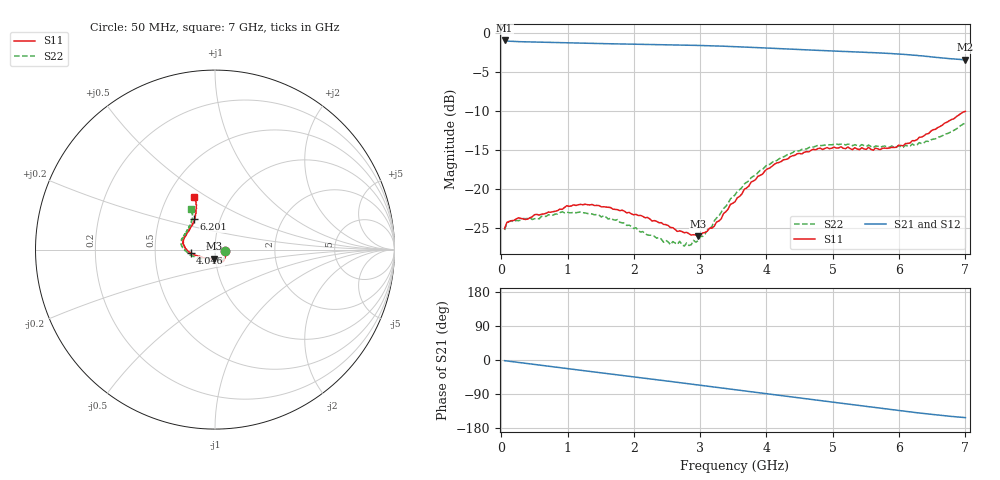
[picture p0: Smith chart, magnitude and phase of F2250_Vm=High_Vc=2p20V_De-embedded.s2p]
! Integrated Device Technology
! Corporate Headquarters
! 6024 Silver Creek Valley Road
! San Jose, CA 95138  USA
! Phone:  1-408-284-8200
! Toll Free:  1-800-223-1366
! Webpage:  http://www.idt.com/
! Timing and RF Division
! 515 Groton Road, Suite 102
! Westford, MA 01886-6024
! Device:  F2250
! Description: Voltage Variable RF Attenuator
! Frequency:  50.0 -  6000.00 MHz
! Package:  3x3 mm Thin QFN Plastic Package: 16 pin
! Ports:  2 RF, 3 DC
!  Pin  1  = GND
!  Pin  2  = NC
!  Pin  3  = RF1  = Port 1
!  Pin  4  = NC
!  Pin  5  = GND
!  Pin  6  = GND
!  Pin  7  = GND
!  Pin  8  = GND
!  Pin  9  = NC
!  Pin 10  = RF2  = Port 2
!  Pin 11  = NC
!  Pin 12  = GND
!  Pin 13  = GND
!  Pin 14  = VCNTRL
!  Pin 15  = VDD
!  Pin 16  = VMODE
! Vcntrl:  2.200 Volts
! Vmode:  +3.300 Volts
! Vdd:  +3.30  Volts
! Current:  1.317 mA
! Data:  The device was measured on a the F2250 evaluation board which has
!  individual transmission lines to the RF pins.  Data was collected
!  using a calibrated network analyzer.  The evaluation board was
!  de-embedded using a TRL calibration technique.
!  The reference plane is the edge of the package pin.
! Misc:  SN 10
!  Action Tracker AT0258
! Date Measured:  2014-11-26
! Date:  2015-10-15  MJV
! Note:
!  Integrated Device Technology supplies this data as a sample of measured
!  data at the package pin for this product.  Your particular data for this
!  product may vary.
!  Data was taken at 25 degrees C.
!  Integrated Device Technology reserves the right to change this data at anytime.
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# GHz S dB R 50
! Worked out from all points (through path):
!   201 points, 50 MHz to 7 GHz, reference 50 ohm
!   highest |S21| = -0.93 dB at 50 MHz (marker M1); lowest = -3.4 dB at 7 GHz (marker M2)
!   group delay of S21, straight-line fit = 61.1 ps
!   lowest |S11| = -26.0 dB at 2.969 GHz (marker M3), VSWR 1.11, Z = 49.4 - j4.96 ohm
!   |S11| at or under -10 dB: start of sweep to end of sweep
!   |S22| runs from -27.3 to -11.5 dB; largest |S21 - S12| = 0.0019
!   S11 on the Smith chart (normalised r, x): 50 MHz: 1.12, -0.02; 4.046 GHz: 0.76, -0.03; 6.201 GHz: 0.75, +0.27; 7 GHz: 0.68, +0.44
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0.05  -25.02 -9.9  -0.93 -1.8  -0.93 -1.8  -25.20 -10.3
0.08475  -24.23 -9.1  -1.00 -2.5  -1.00 -2.5  -24.28 -9.2
0.1195  -24.12 -9.6  -1.03 -3.2  -1.03 -3.2  -24.09 -8.5
0.91875  -22.56 -48.1  -1.21 -21.0  -1.21 -21.1  -22.87 -49.8
1.2315  -21.97 -55.9  -1.28 -27.9  -1.28 -27.9  -22.99 -60.3
1.75275  -22.59 -62.8  -1.37 -39.1  -1.37 -39.1  -23.87 -67.1
2.37825  -24.27 -62.8  -1.46 -52.8  -1.46 -52.8  -26.16 -67.8
2.552  -24.89 -67.4  -1.49 -56.6  -1.49 -56.7  -27.08 -74.4
2.691  -25.31 -75.0  -1.51 -59.7  -1.51 -59.8  -26.65 -81.7
2.7605  -25.55 -77.0  -1.53 -61.3  -1.53 -61.3  -27.27 -86.1
2.969  -25.99 -94.1  -1.57 -66.0  -1.57 -66.0  -26.58 -104.7
3.21225  -24.72 -123.9  -1.62 -71.5  -1.62 -71.5  -24.04 -129.2
3.525  -21.59 -149.9  -1.72 -78.5  -1.72 -78.5  -20.70 -147.8
3.76825  -19.06 -162.6  -1.81 -84.0  -1.81 -84.0  -18.50 -159.0
4.04625  -17.28 -172.4  -1.92 -90.2  -1.92 -90.2  -16.80 -169.4
4.4285  -15.64 177.3  -2.07 -98.6  -2.07 -98.6  -15.09 179.1
4.7065  -14.87 170.3  -2.17 -104.8  -2.17 -104.8  -14.59 173.3
5.054  -14.71 162.1  -2.30 -112.5  -2.29 -112.5  -14.19 166.3
5.85325  -14.71 136.0  -2.60 -130.0  -2.60 -130.1  -14.59 147.4
6.20075  -13.75 124.4  -2.80 -137.7  -2.81 -137.8  -14.19 138.4
6.54825  -12.31 116.2  -3.08 -144.7  -3.08 -144.8  -13.53 127.0
7  -10.00 111.3  -3.40 -152.1  -3.41 -152.2  -11.51 120.8
